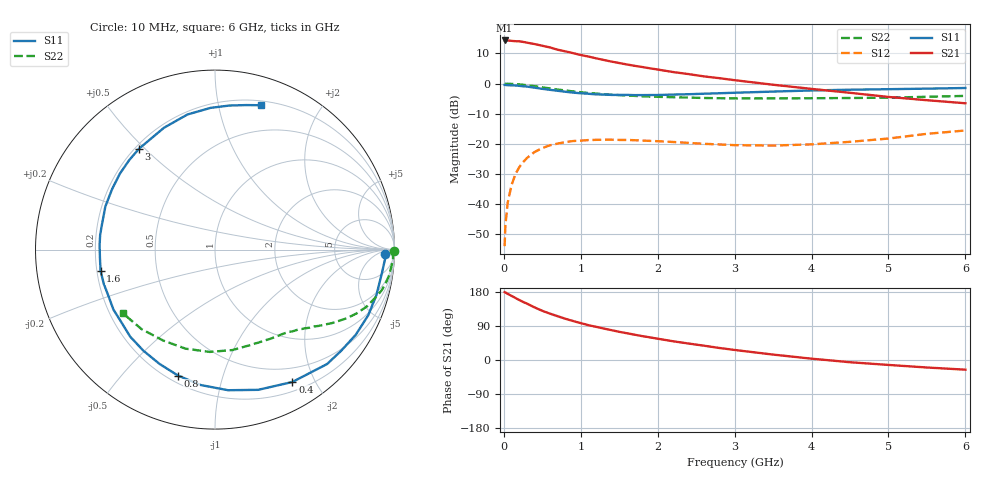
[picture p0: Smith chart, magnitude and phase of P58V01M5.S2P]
! SIEMENS Small Signal Semiconductors
! BFP183
! Si NPN RF Bipolar Junction Transistor in SOT143
! VCE = 8 V  IC = 1.5 mA
! Common Emitter S-Parameters:  March  1996
# GHz  S  MA  R  50
!  f  S11  S21  S12  S22
! GHz  MAG  ANG  MAG  ANG  MAG  ANG  MAG  ANG
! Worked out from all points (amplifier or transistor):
!   36 points, 10 MHz to 6 GHz, reference 50 ohm
!   highest |S21| = 14.3 dB at 10 MHz (marker M1)
!   |S21| within 3 dB of that: start of sweep to 690.2 MHz
!   unconditionally stable (mu >= 1): 2.345 GHz to 5.924 GHz
!   at 250 MHz: K = 0.10, MSG = 20.0 dB, |S12| = -26.1 dB
!   at 1.4 GHz: K = 0.59, MSG = 13.0 dB, |S12| = -18.6 dB
!   at 6 GHz: K = 0.98, MSG = 4.5 dB, |S12| = -15.6 dB
!   S11 on the Smith chart (normalised r, x): 10 MHz: 30, -16; 400 MHz: 0.31, -1.70; 800 MHz: 0.24, -0.72; 1.6 GHz: 0.21, -0.09; 3 GHz: 0.22, +0.48; 6 GHz: 0.24, +1.34
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0.01  0.9486 -1.6  5.193 179.1  0.002 92.8  0.9998 -0.6
0.02  0.9487 -3.2  5.184 178.4  0.0044 89.0  0.9901 -1.1
0.05  0.9393 -7.9  5.17 174.6  0.0106 88.4  0.9933 -2.8
0.1  0.9344 -15.7  5.119 169.2  0.0206 80.7  0.9867 -5.6
0.2  0.9167 -31.1  5.03 158.4  0.0409 71.7  0.9696 -11.1
0.25  0.901 -38.8  4.915 153.2  0.0495 67.6  0.9556 -13.8
0.4  0.8543 -59.7  4.526 138.8  0.0732 56.0  0.9048 -20.4
0.5  0.8175 -72.9  4.239 129.8  0.085 48.9  0.8658 -24.2
0.6  0.7868 -84.7  3.979 122.3  0.0945 43.0  0.8293 -27.4
0.7  0.7587 -96.0  3.645 115.5  0.1009 37.5  0.7951 -30.0
0.8  0.7316 -106.3  3.424 108.8  0.1068 32.9  0.7678 -32.3
0.9  0.7079 -115.9  3.199 102.9  0.1112 28.8  0.7408 -34.3
1.1  0.6772 -134.2  2.805 91.9  0.1154 21.8  0.6977 -37.9
1.3  0.6572 -149.4  2.461 83.0  0.1169 16.3  0.667 -41.1
1.6  0.6485 -169.5  2.075 70.6  0.1159 10.4  0.635 -45.3
1.8  0.6433 178.0  1.883 63.0  0.1132 7.9  0.615 -48.2
2.2  0.6565 158.5  1.553 49.4  0.1072 4.3  0.5931 -54.6
3  0.7037 127.0  1.138 26.5  0.095 6.0  0.5672 -69.4
3.5  0.7361 112.7  0.956 14.3  0.0935 11.5  0.5681 -80.1
4.5  0.7901 91.8  0.702 -5.9  0.1079 22.4  0.5757 -106.5
5.5  0.8235 77.9  0.529 -19.8  0.1465 25.7  0.6033 -132.8
6  0.8443 72.3  0.471 -25.5  0.1664 22.8  0.6241 -145.4
